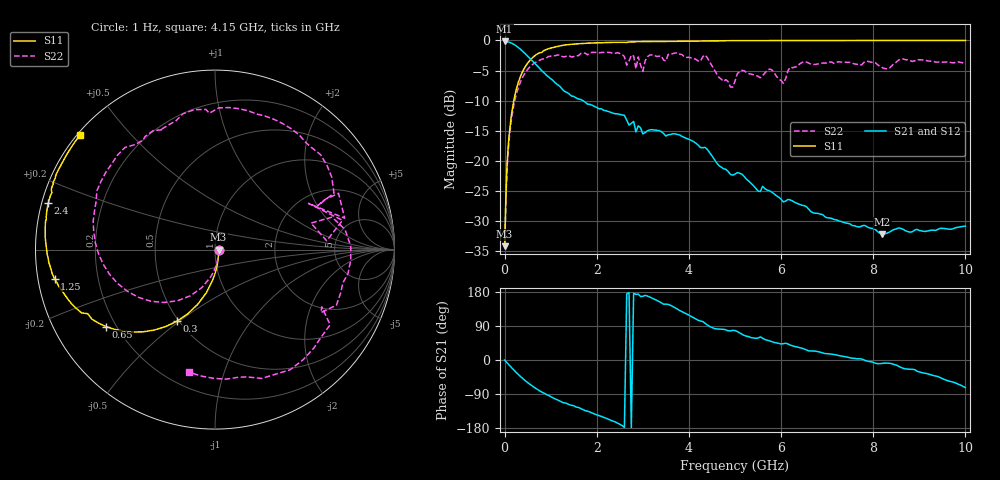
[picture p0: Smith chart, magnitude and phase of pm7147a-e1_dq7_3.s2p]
# GHz S DB R 50
! S-Parameters data
! Freq  dbS11  angS11  dbS21  angS21  dbS12  angS12  dbS22  angS22
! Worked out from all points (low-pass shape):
!   279 points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, 1 Hz to 10 GHz, reference 50 ohm
!   highest |S21| = -0.17 dB at 15.85 kHz (marker M1); lowest = -32.1 dB at 8.2 GHz (marker M2)
!   |S21| within 3 dB of the highest: start of sweep to 573 MHz
!   lowest |S11| = -34.1 dB at 15.85 kHz (marker M3), VSWR 1.04, Z = 52 - j0.00256 ohm
!   |S11| at or under -10 dB: start of sweep to 198.1 MHz
!   |S22| runs from -34.1 to -2.0 dB; largest |S21 - S12| = 5.5e-13
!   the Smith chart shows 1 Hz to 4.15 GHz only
!   S11 on the Smith chart (normalised r, x): 1 Hz: 1.04, -0.00; 300 MHz: 0.49, -0.49; 650 MHz: 0.16, -0.31; 1.25 GHz: 0.05, -0.09; 2.4 GHz: 0.02, +0.14; 4.15 GHz: 0.01, +0.37
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1e-09  -34.12 -0.0  -0.17 -0.0  -0.17 -0.0  -34.12 -0.0
1.58489e-05  -34.12 -0.1  -0.17 -0.0  -0.17 -0.0  -34.12 -0.1
0.03981072  -23.17 -77.3  -0.20 -5.4  -0.20 -5.4  -23.88 -78.1
0.1  -15.57 -93.9  -0.30 -13.5  -0.30 -13.5  -16.32 -98.8
0.3  -6.90 -118.0  -1.19 -38.5  -1.19 -38.5  -7.76 -133.9
0.65  -2.57 -144.8  -3.77 -72.7  -3.77 -72.7  -3.74 -178.1
1.25  -0.83 -169.8  -8.08 -111.7  -8.08 -111.7  -2.68 127.1
1.7  -0.51 178.1  -9.99 -130.9  -9.99 -130.9  -2.07 98.5
2.4  -0.32 164.4  -12.16 -163.3  -12.16 -163.3  -2.13 46.8
3.05  -0.18 154.3  -15.28 170.6  -15.28 170.6  -3.39 15.5
3.35  -0.18 149.9  -14.96 154.2  -14.96 154.2  -2.61 -18.8
3.75  -0.15 144.6  -15.59 134.4  -15.59 134.4  -2.05 -58.0
4.15  -0.12 139.7  -17.03 108.2  -17.03 108.2  -3.12 -101.9
4.4  -0.09 136.7  -18.09 92.3  -18.09 92.3  -2.88 -135.3
4.65  -0.06 133.7  -20.76 81.6  -20.76 81.6  -6.12 -159.1
5.05  -0.04 129.0  -21.92 75.0  -21.92 75.0  -5.51 -166.5
5.8  -0.03 121.2  -25.17 48.4  -25.17 48.4  -4.88 135.6
6.7  -0.01 112.6  -28.59 23.9  -28.59 23.9  -3.99 98.3
8.2  -0.00 100.2  -32.12 -8.8  -32.12 -8.8  -4.53 38.8
8.35  -0.01 99.1  -31.80 -8.7  -31.80 -8.7  -4.59 39.9
9.1  -0.01 93.8  -31.67 -34.6  -31.67 -34.6  -3.25 3.9
10  -0.01 88.1  -30.80 -72.9  -30.80 -72.9  -3.88 -53.3
